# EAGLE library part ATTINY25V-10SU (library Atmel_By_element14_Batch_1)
8-bit Microcontroller with In-System Programmable Flash
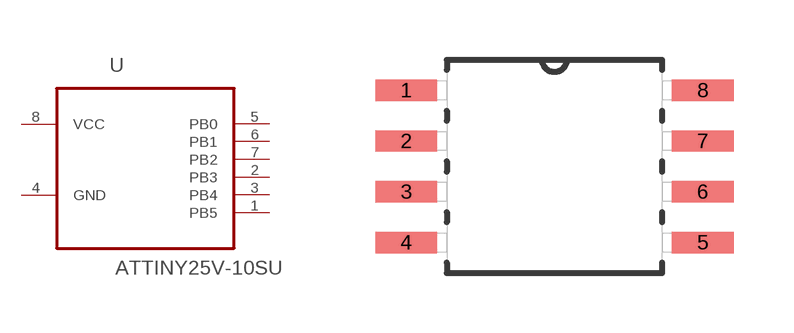
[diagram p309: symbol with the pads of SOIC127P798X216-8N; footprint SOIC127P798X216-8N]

Designator prefix U

## ATTINY25V-10SU (MPN: ATTINY25V-10SU; OC_FARNELL: 1455145; OC_NEWARK: 58M3781; PACKAGE: SOIC-8; SUPPLIER: Atmel)  [SOIC127P798X216-8N]
1  PB5
2  PB3
3  PB4
4  GND  pas
5  PB0
6  PB1
7  PB2
8  VCC  pwr

## Footprint SOIC127P798X216-8N (pad centres in mm)
smd 1.549 x 0.533: 1 -3.708,1.905; 2 -3.708,0.635; 3 -3.708,-0.635; 4 -3.708,-1.905; 5 3.708,-1.905; 6 3.708,-0.635; 7 3.708,0.635; 8 3.708,1.905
